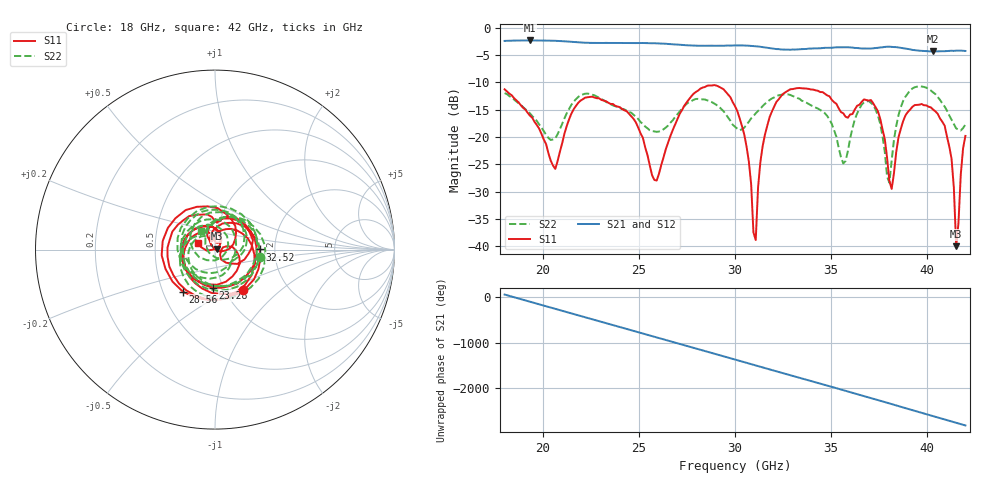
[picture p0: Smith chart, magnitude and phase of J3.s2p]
!Agilent Technologies,N5230A,US43500212,A.07.50.67
!Agilent N5230A: A.07.50.67
!Date: Monday, September 22, 2025 05:53:53
!Correction: S11(Full 2 Port(1,2))
!S21(Full 2 Port(1,2))
!S12(Full 2 Port(1,2))
!S22(Full 2 Port(1,2))
!S2P File: Measurements: S11, S21, S12, S22:
# Hz S  dB  R 50
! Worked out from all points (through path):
!   201 points, 18 GHz to 42 GHz, reference 50 ohm
!   highest |S21| = -2.33 dB at 19.32 GHz (marker M1); lowest = -4.3 dB at 40.32 GHz (marker M2)
!   lowest |S11| = -40.0 dB at 41.52 GHz (marker M3), VSWR 1.02, Z = 50.8 + j0.56 ohm
!   |S11| at or under -10 dB: start of sweep to end of sweep
!   |S22| runs from -28.4 to -10.7 dB; largest |S21 - S12| = 0.0077
!   S11 on the Smith chart (normalised r, x): 18 GHz: 1.21, -0.59; 23.28 GHz: 0.89, -0.40; 28.56 GHz: 0.63, -0.33; 32.52 GHz: 1.67, +0.00; 42 GHz: 0.82, +0.06
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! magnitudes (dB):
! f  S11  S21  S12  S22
! 18 GHz  -11.3  -2.4  -2.4  -12.0
! 19.32 GHz  -16.1  -2.3  -2.3  -15.6
! 20.64 GHz  -25.8  -2.4  -2.4  -20.2
! 22.08 GHz  -13.1  -2.7  -2.7  -12.2
! 23.28 GHz  -13.4  -2.8  -2.8  -13.6
! 26.04 GHz  -26.7  -2.9  -2.9  -19.0
! 28.56 GHz  -10.6  -3.3  -3.3  -13.3
! 30 GHz  -14.3  -3.2  -3.2  -18.1
! 30.6 GHz  -21.7  -3.3  -3.3  -17.7
! 31.08 GHz  -38.8  -3.4  -3.4  -15.7
! 31.44 GHz  -21.7  -3.6  -3.5  -14.3
! 32.52 GHz  -12.1  -4.0  -4.0  -12.2
! 34.08 GHz  -11.3  -3.8  -3.8  -14.4
! 35.64 GHz  -15.7  -3.6  -3.6  -24.8
! 36.48 GHz  -14.1  -3.8  -3.8  -14.8
! 37.2 GHz  -13.8  -3.8  -3.8  -14.1
! 38.04 GHz  -28.0  -3.5  -3.5  -28.4
! 38.76 GHz  -17.1  -3.7  -3.8  -13.4
! 40.32 GHz  -15.0  -4.3  -4.3  -11.8
! 41.28 GHz  -24.0  -4.2  -4.2  -16.8
! 41.52 GHz  -40.0  -4.2  -4.2  -18.4
! 42 GHz  -19.8  -4.3  -4.2  -17.7
